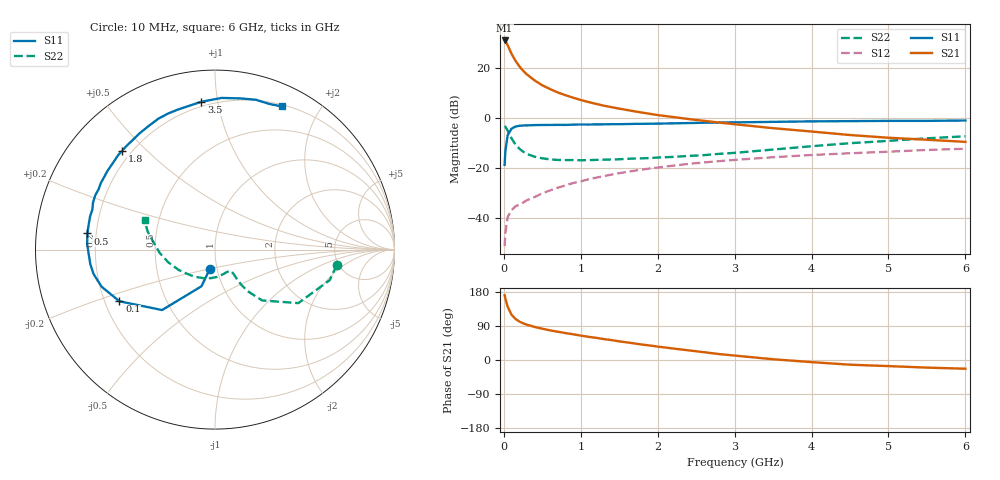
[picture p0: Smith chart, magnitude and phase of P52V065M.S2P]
! SIEMENS Small Signal Semiconductors
! BFP183
! Si NPN RF Bipolar Junction Transistor in SOT143
! VCE = 2 V  IC = 65 mA
! Common Emitter S-Parameters:  March  1996
# GHz  S  MA  R  50
!  f  S11  S21  S12  S22
! GHz  MAG  ANG  MAG  ANG  MAG  ANG  MAG  ANG
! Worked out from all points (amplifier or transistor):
!   36 points, 10 MHz to 6 GHz, reference 50 ohm
!   highest |S21| = 30.9 dB at 10 MHz (marker M1)
!   |S21| within 3 dB of that: start of sweep to 66.02 MHz
!   unconditionally stable (mu >= 1): start of sweep to 39.71 MHz; 144.4 MHz to end of sweep
!   at 250 MHz: K = 1.34, MAG = 22.9 dB, |S12| = -33.9 dB
!   at 1.4 GHz: K = 1.83, MAG = 8.2 dB, |S12| = -22.7 dB
!   at 6 GHz: K = 1.43, MAG = -2.5 dB, |S12| = -12.4 dB
!   S11 on the Smith chart (normalised r, x): 10 MHz: 0.92, -0.21; 100 MHz: 0.26, -0.24; 500 MHz: 0.17, +0.06; 1.8 GHz: 0.16, +0.42; 3.5 GHz: 0.17, +0.90; 6 GHz: 0.22, +1.55
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0.01  0.1142 -105.4  35.12 171.0  0.0027 62.1  0.6838 -7.2
0.02  0.2175 -110.2  34.12 162.3  0.005 60.3  0.6615 -14.9
0.05  0.4476 -131.2  28.2 140.3  0.0103 56.7  0.5518 -32.7
0.1  0.6055 -151.6  19.02 119.6  0.0142 45.4  0.387 -47.1
0.15  0.6648 -161.9  13.86 108.6  0.0169 44.7  0.2939 -51.9
0.2  0.6897 -168.5  10.75 101.7  0.0183 46.7  0.2416 -53.3
0.25  0.6994 -173.3  8.724 96.8  0.0201 48.2  0.2102 -53.5
0.3  0.7029 -177.1  7.349 93.2  0.0224 51.4  0.1883 -53.0
0.4  0.7128 177.6  5.578 87.2  0.0259 54.7  0.1661 -52.6
0.5  0.7169 172.8  4.452 82.6  0.0308 56.5  0.1543 -53.1
0.6  0.7174 169.1  3.747 78.3  0.0351 59.2  0.147 -54.4
0.7  0.7202 165.1  3.204 74.6  0.0398 60.7  0.1432 -56.1
0.9  0.7283 159.0  2.519 67.9  0.0494 61.4  0.1423 -60.7
1.1  0.7307 152.4  2.061 61.2  0.0587 61.4  0.1418 -66.3
1.5  0.744 141.3  1.519 49.2  0.0778 59.4  0.1477 -79.2
1.8  0.7559 133.1  1.266 40.7  0.0919 57.0  0.1543 -90.2
2.2  0.7717 123.2  1.034 30.3  0.1101 52.9  0.1647 -104.7
2.8  0.802 109.0  0.8 15.6  0.1355 46.2  0.1895 -127.1
3.5  0.8272 95.3  0.618 2.0  0.1622 38.7  0.231 -150.3
4.5  0.8545 80.3  0.451 -12.4  0.1948 27.7  0.3095 -176.8
5.5  0.8659 69.6  0.363 -20.1  0.2269 18.0  0.3873 165.2
6  0.8805 64.9  0.329 -23.0  0.2394 12.6  0.425 157.5
